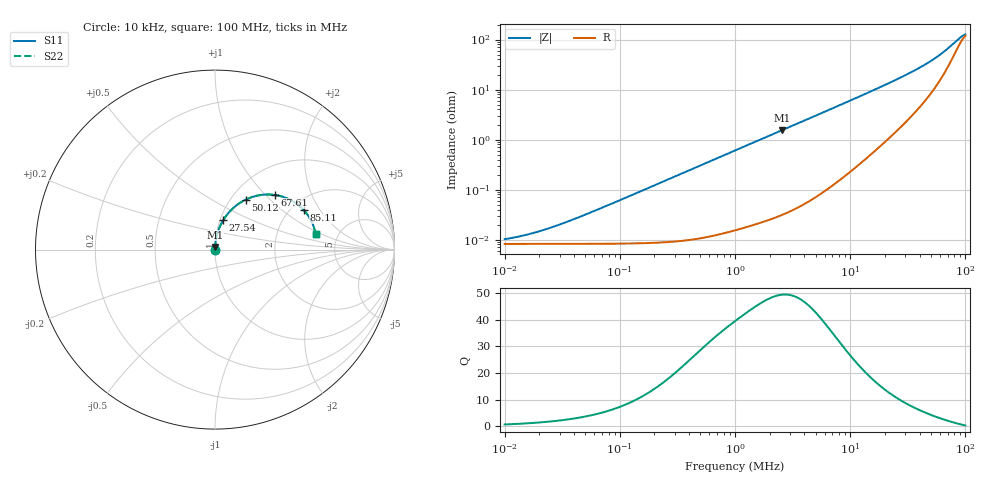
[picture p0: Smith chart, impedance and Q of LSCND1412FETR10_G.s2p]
! LSCND1412FETR10_G  S-PARAMETER MODEL  ( Standard Model )
! Model Generated by TAIYO YUDEN Corporation (http://www.ty-top.com)
! Version 1.0
! TAIYO YUDEN Control No. 231201
! Copyright(c) 2023 TAIYO YUDEN CO.,LTD. All Rights Reserved.
! Product Description (link to TY-COMPAS)
! https://ds.yuden.co.jp/TYCOMPAS/or/detail?pn=LSCND1412FETR10MG&u=M
! Products Name : Inductors
! Characteristics :
!  Inductance : 0.1 [uH] , SRF(min) : - [Hz] , DC Resistance(max) : 10 [mOhm]
!  Rated Current : Saturation  6.8 [A] (dL = 30 [%]), Temp Rise  6.7 [A] (dT = 40 [degC])
!  Case Size : 1.4 x 1.2 / 0.055 x 0.047 [mm/inch] , Thickness : 0.65 / 0.026 [mm/inch]
!  (Conditions: Temperature = 25 [degC] , DC Bias Current = 0 [A])
! External Node Assignments :
!  1  o---GGG---o  2
! GND o---------o GND
! Frequency Range : 10kHz  -  100MHz  [ 402 STEP ]
# MHz S RI R 50
! Freq[MHz].  S11 Real  S11 Imag  S21 Real  S21 Imag  S12 Real  S12 Imag  S22 Real  S22 Imag
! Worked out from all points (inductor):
!   401 points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, 10 kHz to 100 MHz, reference 50 ohm
!   read as one part in series: L = 96.8 nH near 40.74 kHz
!   highest Q = 49.3 at 2.57 MHz (marker M1), where L = 95.5 nH
!   S11 on the Smith chart (normalised r, x): 10 kHz: 1.00, +0.00; 27.54 MHz: 1.04, +0.35; 50.12 MHz: 1.17, +0.73; 67.61 MHz: 1.48, +1.13; 85.11 MHz: 2.33, +1.45; 100 MHz: 3.38, +0.88
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0.01  8.2e-05 6.08e-05  0.9999 -6.08e-05  0.9999 -6.08e-05  8.2e-05 6.08e-05
0.013804  8.2e-05 8.39e-05  0.9999 -8.39e-05  0.9999 -8.39e-05  8.2e-05 8.39e-05
0.019953  8.2e-05 0.000121  0.9999 -0.000121  0.9999 -0.000121  8.2e-05 0.000121
0.029512  8.21e-05 0.000179  0.9999 -0.000179  0.9999 -0.000179  8.21e-05 0.000179
0.046774  8.23e-05 0.000284  0.9999 -0.000284  0.9999 -0.000284  8.23e-05 0.000284
0.085114  8.31e-05 0.000517  0.9999 -0.000517  0.9999 -0.000517  8.31e-05 0.000517
0.218776  8.89e-05 0.00133  0.9999 -0.00133  0.9999 -0.00133  8.89e-05 0.00133
1  0.000189 0.00603  0.9998 -0.00603  0.9998 -0.00603  0.000189 0.00603
2.570396  0.00055 0.0154  0.9995 -0.0154  0.9995 -0.0154  0.00055 0.0154
4.677351  0.00142 0.028  0.9986 -0.028  0.9986 -0.028  0.00142 0.028
11.22019  0.00733 0.067  0.9927 -0.067  0.9927 -0.067  0.00733 0.067
21.87762  0.0282 0.1304  0.9718 -0.1304  0.9718 -0.1304  0.0282 0.1304
27.54229  0.0456 0.1635  0.9544 -0.1635  0.9544 -0.1635  0.0456 0.1635
38.90451  0.0963 0.2266  0.9037 -0.2266  0.9037 -0.2266  0.0963 0.2266
44.66836  0.1313 0.2551  0.8687 -0.2551  0.8687 -0.2551  0.1313 0.2551
50.11872  0.1705 0.2782  0.8295 -0.2782  0.8295 -0.2782  0.1705 0.2782
58.88437  0.246 0.3027  0.754 -0.3027  0.754 -0.3027  0.246 0.3027
67.6083  0.3323 0.3045  0.6677 -0.3045  0.6677 -0.3045  0.3323 0.3045
75.85776  0.4152 0.2793  0.5848 -0.2793  0.5848 -0.2793  0.4152 0.2793
85.1138  0.4946 0.2202  0.5054 -0.2202  0.5054 -0.2202  0.4946 0.2202
93.32543  0.5414 0.1493  0.4586 -0.1493  0.4586 -0.1493  0.5414 0.1493
100  0.5605 0.0879  0.4395 -0.0879  0.4395 -0.0879  0.5605 0.0879
